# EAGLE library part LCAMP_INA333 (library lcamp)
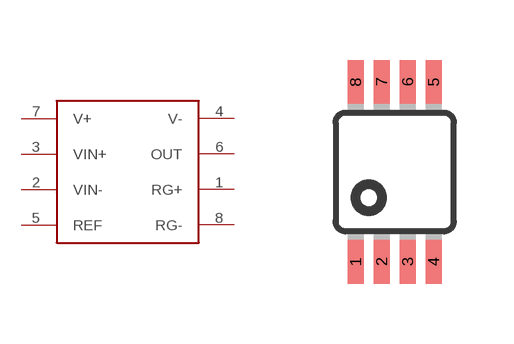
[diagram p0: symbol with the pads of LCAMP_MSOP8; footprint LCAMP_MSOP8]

Designator prefix U

## LCAMP_INA333MSOP8  [LCAMP_MSOP8]
1  RG+
2  VIN-
3  VIN+
4  V-
5  REF
6  OUT
7  V+
8  RG-

## Footprint LCAMP_MSOP8 (pad centres in mm)
8M, 8-Lead, 0.118" Wide, Miniature Small Outline Package MSOP 8M-Package doc1097.pdf
smd 0.4 x 1.1: 1 -0.975,-2.25; 2 -0.325,-2.25; 3 0.325,-2.25; 4 0.975,-2.25; 5 0.975,2.25; 6 0.325,2.25; 7 -0.325,2.25; 8 -0.975,2.25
